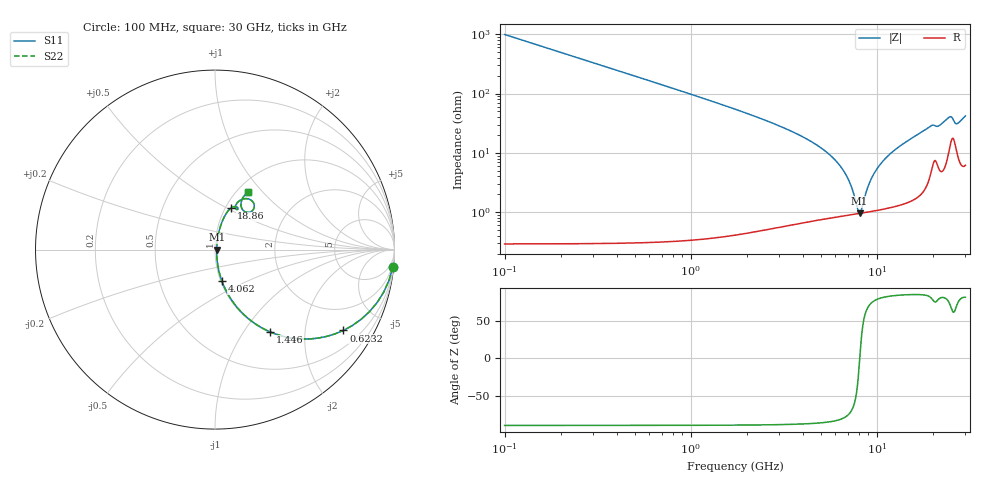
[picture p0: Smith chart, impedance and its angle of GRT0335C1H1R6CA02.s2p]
!Murata Part Number: GRT0335C1H1R6CA02
!These Parameters are Measured in Series Mode Connection
!Data Generated on Jun 19, 2026
!  o--ll--o
!Port1  Port2
!  o------o
!Operation Temp=25[degC], DC Bias Voltage=0[V]
!Freq. Start=100[MHz] Stop=30[GHz] 401[Steps]
# Hz S RI R 50
!Freq.(Hz) S11(Real) S11(Imag) S21(Real) S21(Imag) S12(Real) S12(Imag) S22(Real) S22(Imag)
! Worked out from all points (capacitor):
!   401 points, 100 MHz to 30 GHz, reference 50 ohm
!   read as one part in series: C = 1.6 pF near 249.5 MHz
!   lowest |Z| = 951 mohm at 8.098 GHz (marker M1)
!   series resonance near 8.114 GHz, so ESL is about 240 pH
!   S11 on the Smith chart (normalised r, x): 100 MHz: 1, -20; 623.2 MHz: 1.01, -3.17; 1.446 GHz: 1.01, -1.33; 4.062 GHz: 1.01, -0.36; 18.86 GHz: 1.06, +0.52; 30 GHz: 1.12, +0.83
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1e8  0.99 -0.0995  0.01 0.0995  0.01 0.0995  0.99 -0.0995
3.99e8  0.8605 -0.3459  0.1395 0.3459  0.1395 0.3459  0.8605 -0.3459
6.2325e8  0.7151 -0.4504  0.2849 0.4504  0.2849 0.4504  0.7151 -0.4504
9.97e8  0.4907 -0.4982  0.5093 0.4982  0.5093 0.4982  0.4907 -0.4982
1.4455e9  0.3075 -0.4586  0.6925 0.4586  0.6925 0.4586  0.3075 -0.4586
2.41725e9  0.1255 -0.3248  0.8745 0.3248  0.8745 0.3248  0.1255 -0.3248
4.06175e9  0.0381 -0.174  0.9619 0.174  0.9619 0.174  0.0381 -0.174
5.10825e9  0.0206 -0.1133  0.9794 0.1133  0.9794 0.1133  0.0206 -0.1133
6.8275e9  0.0104 -0.0414  0.9896 0.0414  0.9896 0.0414  0.0104 -0.0414
7.276e9  0.00961 -0.0261  0.9904 0.0261  0.9904 0.0261  0.00961 -0.0261
8.09825e9  0.00941 -0.000461  0.9906 0.000461  0.9906 0.000461  0.00941 -0.000461
8.24775e9  0.00951 0.00392  0.9905 -0.00392  0.9905 -0.00392  0.00951 0.00392
9.14475e9  0.0109 0.0287  0.9891 -0.0287  0.9891 -0.0287  0.0109 0.0287
1.01165e10  0.0135 0.0533  0.9865 -0.0533  0.9865 -0.0533  0.0135 0.0533
1.206e10  0.0216 0.0975  0.9784 -0.0975  0.9784 -0.0975  0.0216 0.0975
1.505e10  0.0408 0.1581  0.9592 -0.1581  0.9592 -0.1581  0.0408 0.1581
1.886225e10  0.0887 0.2311  0.9113 -0.2311  0.9113 -0.2311  0.0887 0.2311
2.005825e10  0.1228 0.2371  0.8772 -0.2371  0.8772 -0.2371  0.1228 0.2371
2.245025e10  0.1229 0.2593  0.8771 -0.2593  0.8771 -0.2593  0.1229 0.2593
2.50665e10  0.2155 0.2581  0.7845 -0.2581  0.7845 -0.2581  0.2155 0.2581
2.678575e10  0.1582 0.2175  0.8418 -0.2175  0.8418 -0.2175  0.1582 0.2175
3e10  0.1831 0.3194  0.8169 -0.3194  0.8169 -0.3194  0.1831 0.3194
